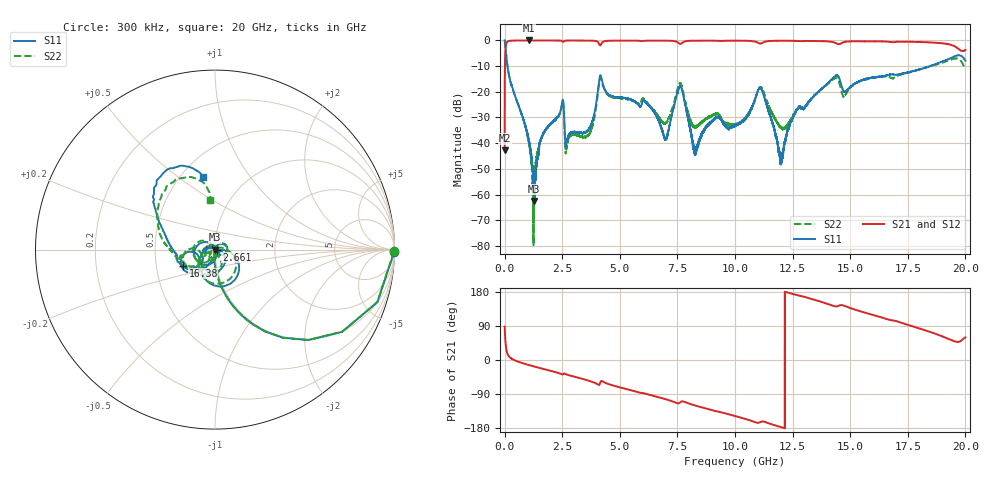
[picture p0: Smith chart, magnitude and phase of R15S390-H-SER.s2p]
!{R15S390}
!Johanson Technology Inc.
!www.johansontechnology.com
!Test Board Conditions:
!Substrate Type  RO4350B
!Substrate Thickness  20 mil
!Substrate Dk  3.66
!TL Type: GCPW
!TL Trace Width  34 mil
!TL Gap  10 mil
!Electrode orientation  Horizontal
!DUT TOPOLOGY	SERIES
!Mounting Pad LxW  26x52 mil
! Created Sat Feb  6 14:27:42 2021
# hz S ma R 50
! 2 Port Network Data from SP1.SP block
! freq  magS11  angS11  magS21  angS21  magS12  angS12  magS22  angS22
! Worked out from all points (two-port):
!   20001 points, 300 kHz to 20 GHz, reference 50 ohm
!   highest |S21| = 0.00 dB at 1.066 GHz (marker M1); lowest = -42.8 dB at 300 kHz (marker M2)
!   |S21| within 3 dB of the highest: 41.59 MHz to 19.66 GHz (19.62 GHz wide, 199 % of centre)
!   lowest |S11| = -62.5 dB at 1.283 GHz (marker M3), VSWR 1.00, Z = 49.9 + j0.016 ohm
!   |S11| at or under -10 dB: 123.1 MHz to 18.46 GHz (18.34 GHz wide, 197 % of centre)
!   |S22| runs from -80.1 to 0.0 dB; largest |S21 - S12| = 0.015
!   S11 on the Smith chart (normalised r, x): 300 kHz: open; 2.661 GHz: 1.02, +0.00; 16.38 GHz: 0.69, -0.13; 20 GHz: 0.65, +0.61
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300000  0.9985 -0.7  0.007232 88.3  0.007264 89.6  0.9976 -0.6
1.303e8  0.3008 -74.1  0.9526 15.6  0.9525 15.6  0.301 -74.2
1.0663e9  0.01058 -105.6  0.9997 -13.5  0.9985 -13.6  0.00948 -103.9
1.2833e9  0.0007468 167.6  0.999 -17.1  0.9991 -17.1  0.001464 67.1
1.6003e9  0.0128 77.1  0.9984 -22.3  0.9983 -22.3  0.01294 57.6
2.4673e9  0.05066 43.2  0.9864 -37.1  0.9868 -37.1  0.04969 37.9
2.6613e9  0.00898 3.4  0.9929 -37.6  0.9926 -37.6  0.006661 3.2
3.3343e9  0.01594 12.3  0.9965 -49.1  0.9961 -49.0  0.01361 55.9
3.7623e9  0.02319 -4.2  0.9916 -56.6  0.9923 -56.6  0.01819 40.6
4.1763e9  0.2056 -85.8  0.8268 -56.6  0.8265 -56.6  0.1886 -93.9
6.6673e9  0.02895 143.6  0.9924 -98.0  0.9927 -98.0  0.03324 -147.2
7.0183e9  0.01241 52.7  0.9896 -104.0  0.99 -104.0  0.02507 -94.9
7.6183e9  0.1272 -101.3  0.8561 -112.2  0.8574 -112.1  0.1474 -110.4
8.2623e9  0.005789 83.9  0.9877 -120.0  0.9881 -120.0  0.02057 -108.5
9.1823e9  0.03107 -43.1  0.9858 -135.2  0.9876 -135.2  0.03783 -74.3
1.00003e10  0.02255 -68.6  0.9894 -147.8  0.9892 -147.7  0.0234 -76.8
1.11173e10  0.1183 -165.7  0.8714 -163.5  0.8715 -163.5  0.1232 -175.5
1.20003e10  0.004731 6.6  0.9863 -177.1  0.9865 -177.0  0.02079 166.1
1.33343e10  0.07535 -109.0  0.9798 161.0  0.9802 160.9  0.07515 -120.0
1.63773e10  0.2002 -153.4  0.956 112.1  0.9535 111.9  0.1983 -162.5
1.66673e10  0.2116 -160.2  0.9451 106.4  0.9323 106.4  0.1974 -169.6
2e10  0.403 99.4  0.6519 59.6  0.6469 59.6  0.2752 95.4
